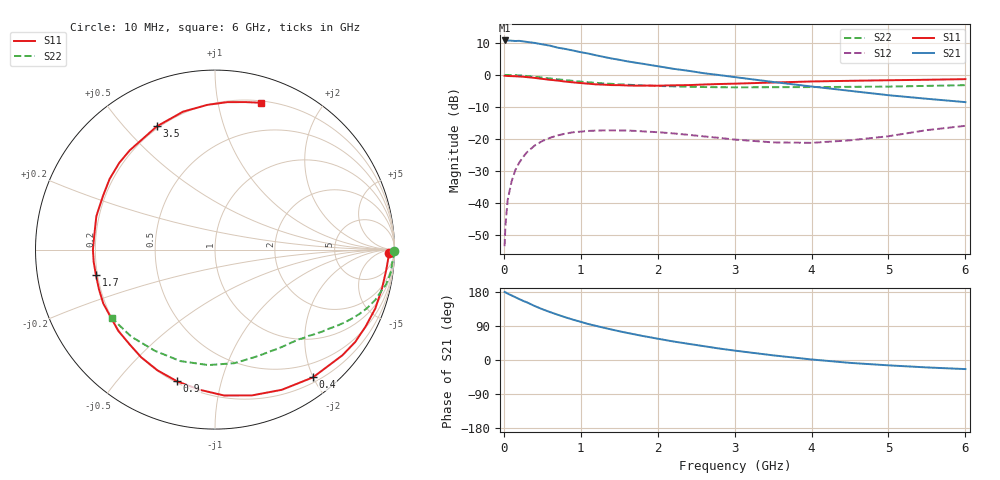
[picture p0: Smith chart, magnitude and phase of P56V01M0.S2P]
! SIEMENS Small Signal Semiconductors
! BFP183
! Si NPN RF Bipolar Junction Transistor in SOT143
! VCE = 6 V  IC = 1 mA
! Common Emitter S-Parameters:  March  1996
# GHz  S  MA  R  50
!  f  S11  S21  S12  S22
! GHz  MAG  ANG  MAG  ANG  MAG  ANG  MAG  ANG
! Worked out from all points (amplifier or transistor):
!   36 points, 10 MHz to 6 GHz, reference 50 ohm
!   highest |S21| = 10.8 dB at 10 MHz (marker M1)
!   |S21| within 3 dB of that: start of sweep to 870.6 MHz
!   unconditionally stable (mu >= 1): 2.504 GHz to end of sweep
!   at 250 MHz: K = 0.10, MSG = 18.1 dB, |S12| = -25.7 dB
!   at 1.4 GHz: K = 0.53, MSG = 11.2 dB, |S12| = -17.3 dB
!   at 6 GHz: K = 1.03, MAG = 2.7 dB, |S12| = -15.9 dB
!   S11 on the Smith chart (normalised r, x): 10 MHz: 44, -29; 400 MHz: 0.27, -2.00; 900 MHz: 0.21, -0.73; 1.7 GHz: 0.19, -0.10; 3.5 GHz: 0.19, +0.62; 6 GHz: 0.22, +1.34
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0.01  0.9688 -1.2  3.452 179.4  0.0021 84.1  0.9995 -0.5
0.02  0.967 -2.7  3.452 178.7  0.0043 85.5  0.9952 -0.9
0.05  0.961 -6.7  3.45 175.2  0.0111 87.2  0.9955 -2.3
0.1  0.9554 -13.1  3.419 170.5  0.0214 81.9  0.9892 -4.7
0.15  0.9514 -20.2  3.386 165.6  0.0326 77.4  0.988 -7.1
0.2  0.9422 -27.1  3.401 160.8  0.0424 74.1  0.9808 -9.2
0.25  0.9355 -33.4  3.342 156.1  0.052 69.3  0.9726 -11.5
0.4  0.8971 -52.5  3.16 142.5  0.0784 58.6  0.9363 -17.4
0.5  0.8653 -64.5  3.004 134.1  0.0924 51.5  0.9074 -21.1
0.6  0.838 -75.8  2.861 126.5  0.1038 45.4  0.8792 -24.2
0.7  0.8145 -86.4  2.664 119.5  0.1133 39.8  0.8525 -26.9
0.9  0.7637 -106.0  2.404 106.4  0.1266 30.1  0.8049 -31.6
1.1  0.7274 -124.4  2.152 94.8  0.133 21.9  0.765 -35.6
1.4  0.6923 -147.1  1.805 80.5  0.1359 12.2  0.724 -40.9
1.7  0.6784 -167.8  1.56 67.7  0.1332 5.0  0.6923 -45.7
2  0.6772 174.6  1.367 56.2  0.1271 -0.3  0.6715 -50.3
2.2  0.6868 164.3  1.246 49.0  0.1218 -3.1  0.6617 -53.9
2.8  0.7198 137.8  0.993 30.3  0.1036 -5.9  0.6414 -65.1
3.5  0.7593 115.3  0.775 12.3  0.088 0.8  0.6419 -80.3
4.5  0.8075 93.0  0.563 -7.6  0.0948 20.1  0.6503 -107.2
5.5  0.8388 78.5  0.423 -19.6  0.1369 27.4  0.6729 -133.9
6  0.8577 72.5  0.375 -24.0  0.1598 24.6  0.6906 -146.6
